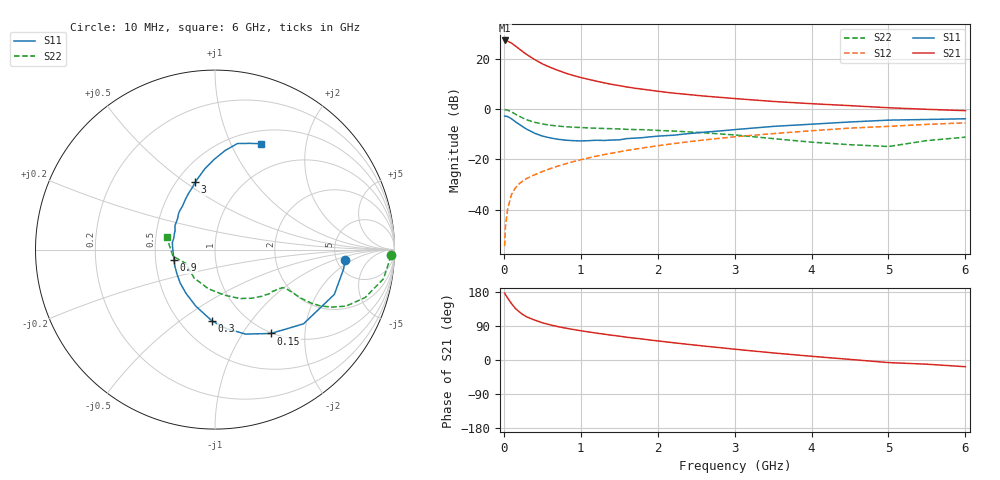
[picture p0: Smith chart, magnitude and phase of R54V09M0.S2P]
! SIEMENS Small Signal Semiconductors
! BFR183
! Si NPN RF Bipolar Junction Transistor in SOT23
! VCE = 4 V  IC = 9 mA
! Common Emitter S-Parameters:  May  1996
# GHz  S  MA  R  50
!  f  S11  S21  S12  S22
! GHz  MAG  ANG  MAG  ANG  MAG  ANG  MAG  ANG
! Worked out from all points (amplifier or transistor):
!   36 points, 10 MHz to 6 GHz, reference 50 ohm
!   highest |S21| = 27.3 dB at 10 MHz (marker M1)
!   |S21| within 3 dB of that: start of sweep to 184.3 MHz
!   unconditionally stable (mu >= 1): 808 MHz to 2.534 GHz
!   at 250 MHz: K = 0.59, MSG = 25.6 dB, |S12| = -28.5 dB
!   at 1.4 GHz: K = 1.05, MAG = 12.3 dB, |S12| = -17.5 dB
!   at 6 GHz: K = 0.89, MSG = 2.4 dB, |S12| = -5.4 dB
!   S11 on the Smith chart (normalised r, x): 10 MHz: 6.02, -1.43; 150 MHz: 0.99, -1.35; 300 MHz: 0.71, -0.66; 900 MHz: 0.62, -0.08; 3 GHz: 0.62, +0.55; 6 GHz: 0.65, +1.31
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0.01  0.7286 -4.4  23.08 176.5  0.0019 83.5  0.9809 -1.9
0.02  0.7241 -8.8  23.04 172.8  0.0045 77.9  0.9722 -4.0
0.05  0.7102 -20.6  22.33 163.3  0.0106 78.9  0.953 -9.8
0.1  0.6435 -40.0  20.41 148.7  0.0203 72.6  0.8785 -17.7
0.15  0.5617 -56.3  17.91 136.1  0.0273 66.9  0.7957 -23.3
0.2  0.5004 -70.2  15.67 127.1  0.033 64.4  0.7235 -26.3
0.25  0.4431 -82.1  13.68 119.4  0.0377 62.3  0.6616 -28.2
0.3  0.3969 -92.6  12.07 113.6  0.0421 62.0  0.6124 -29.1
0.4  0.3323 -108.9  9.648 105.4  0.0497 61.7  0.5476 -29.5
0.5  0.292 -123.7  7.933 98.3  0.0575 62.3  0.5068 -29.1
0.6  0.2688 -136.2  6.782 92.9  0.0656 63.2  0.4798 -28.9
0.7  0.2522 -147.0  5.905 88.2  0.0737 64.0  0.4614 -28.8
0.9  0.2362 -165.7  4.664 80.6  0.0905 64.5  0.4378 -29.1
1.1  0.236 177.7  3.901 74.2  0.1074 64.5  0.424 -30.6
1.3  0.2384 164.9  3.332 68.2  0.1247 64.1  0.4123 -32.1
1.6  0.2602 149.1  2.753 60.1  0.1515 62.6  0.397 -35.8
2.2  0.303 126.6  2.082 45.7  0.2057 58.1  0.3672 -45.2
3  0.3915 106.5  1.622 28.5  0.2821 49.9  0.3072 -62.7
3.5  0.4535 97.2  1.421 18.7  0.3263 43.9  0.2597 -78.1
4.5  0.5554 84.1  1.172 1.6  0.4194 31.7  0.1965 -126.3
5.5  0.6229 71.8  0.991 -11.1  0.4974 19.8  0.2371 -171.1
6  0.6435 66.5  0.932 -17.7  0.5347 12.1  0.2779 165.6
